PROGRAM MAIN

VAR CONSTANT
	cInitSourceFFT			: ST_MA_MultiArray_InitPars := ( eTypeCode := eMA_TypeCode_LREAL, nDims := 1, aDimSizes := [cFFTLength]);	
	cInitSourceSDFT			: ST_MA_MultiArray_InitPars := ( eTypeCode := eMA_TypeCode_LREAL, nDims := 1, aDimSizes := [cOversamples]);
	cInitParsSDFT			: ST_CM_SlidingDFT_InitPars := ( nWindowLength := cFFTLength, nBins := cBins, fDampingFactor := cDampingFactor);
END_VAR

VAR
	(* Input *)
	nInputSelection		: UDINT := 1;						// Switch between hardware and function generator	
	nSample				: UDINT;   
	aEl3632 AT %I*		: ARRAY[1..cOversamples] OF INT;	// Input from hardware e.g. EL3632
	
	(* Signal generation *)
	fbFunctionGenerator	: FB_FunctionGenerator;
	nSetFrequencyBin	: UDINT		:= 32;
	fSetFrequency		: LREAL 	:= nSetFrequencyBin * cResolution;	// Frequency of generated signal in Hz
	fSetAmplitude		: LREAL 	:= 5;								// peak amplitude OF SIN signal in Volts	
    fDC					: LREAL 	:= 1;       						// Amplitude of DC in Volts
	
	(* Source buffers *)	
	aBuffer				: ARRAY[1..cOversamples] OF LREAL;				// local varibale -> to source
	fbSourceFFT			: FB_CMA_Source :=(stInitPars := cInitSourceFFT, nOwnID := eID_SourceFFT, aDestIDs := [eID_FFT], nResultBuffers := 6);
	fbSourceSDFT		: FB_CMA_Source :=(stInitPars := cInitSourceSDFT, nOwnID := eID_SourceSDFT, aDestIDs := [eID_SDFT], nResultBuffers := 10);

	(* Sliding DFT *)
	bConfigured			: BOOL := FALSE;
	aConfParams			: ARRAY[1..cBins] OF UDINT;
	fbSlidingDFT		: FB_CMA_SlidingDFT := (stInitPars := cInitParsSDFT, nOwnID := eID_SDFT, aDestIDs := [eID_SinkSDFT]);
	
	(* Result buffers *)										
	aFFTResult			: ARRAY[1..cFFTResult] OF LCOMPLEX;				// local result variable <- from sink
	aSDFTResult			: ARRAY[1..cBins] OF LCOMPLEX;					// local result variable <- from sink
    
	(* Sinks *)
	fbSink_FFT			: FB_CMA_Sink := (nOwnID := eID_SinkFFT);		// Initialize sink buffers
	fbSink_SDFT			: FB_CMA_Sink := (nOwnID := eID_SinkSDFT);		// Initialize sink buffers
	
	(* post-processing of fft *)
	bCalculateFFT		: BOOL;											// true if fft calculation ready
	bCalculateSDFT		: BOOL;											// true if zoom fft calculation ready
	
	aSpectrumAbsFFT     : ARRAY[1..cFFTResult] OF LREAL; 				// magnitude spectrum
	aSpectrumFFTwin		: ARRAY[1..cFFTResult] OF LCOMPLEX;				// magnitude spectral bins
	aSpectrumAbsFFTwin	: ARRAY[1..cFFTResult] OF LREAL; 				// magnitude spectral bins
	
	aSpectrumAbsSDFT	: ARRAY[1..cBins] OF LREAL; 					// magnitude spectral bins
	aSpectrumSDFTwin	: ARRAY[1..cBins] OF LCOMPLEX;					// magnitude spectral bins
	aSpectrumAbsSDFTwin	: ARRAY[1..cBins] OF LREAL; 					// magnitude spectral bins
	
	(* error monitoring *)
	fbErrHist			: FB_HRErrHist;
END_VAR

(* Input *) 
CASE nInputSelection OF
	0:  (* input from EL3632 *)
		FOR nSample := 1 TO cOversamples DO
			aBuffer[nSample] := INT_TO_LREAL(aEl3632[nSample]);
		END_FOR
	1:  (* signal generator *)	
		fSetFrequency := nSetFrequencyBin * cResolution;
		fbFunctionGenerator(	fFrequency 	:= fSetFrequency,
								fAmplitude 	:= fSetAmplitude,
								eFunction 	:= E_FunctionType.Sine,
								aSignal		:= aBuffer );		
        // add DC to signal
		FOR nSample := 1 TO cOversamples DO
			aBuffer[nSample] := fDC + aBuffer[nSample];
		END_FOR								
END_CASE					

(* Call source to collect data *)
SourceBuffers();

(* Calculate Sliding DFT *)
CalculateSDFT();

(* Push results to sink *)
CollectFFT();

ACTION CalculateSDFT:
// Configure
IF NOT bConfigured THEN
	FOR nSample := 1 TO cBins DO
		aConfParams[nSample] := nSample - 1;
	END_FOR 
	fbSlidingDFT.Configure(pArg := ADR(aConfParams), nArgSize := SIZEOF(aConfParams));
	IF fbSlidingDFT.bError THEN
		fbErrHist.AddError(bErr:=TRUE, hrErrCode:=fbSlidingDFT.hrErrorCode, sErrSource:='MAIN.fbSlidingDFT.Configure'); // error monitoring
		// ToDo: if error
	ELSE
		bConfigured := TRUE;
	END_IF
END_IF

// Call SDFT 
fbSlidingDFT.Call();
IF fbSlidingDFT.bError THEN
	fbErrHist.AddError(bErr:=TRUE, hrErrCode:=fbSlidingDFT.hrErrorCode, sErrSource:='MAIN.fbSlidingDFT'); // error monitoring
	// ToDo: if error
END_IF

// Get SDFT
fbSink_SDFT.Output1DStd(pDataOut 		:= ADR(aSDFTResult), 
						nDataOutSize 	:= SIZEOF(aSDFTResult), 
						eElementType 	:= eMA_TypeCode_LCOMPLEX, 
						nOptionPars		:= 0,
						bNewResult		=> bCalculateSDFT);
IF fbSink_SDFT.bError THEN
	fbErrHist.AddError(bErr:=TRUE, hrErrCode:=fbSink_SDFT.hrErrorCode, sErrSource:='MAIN.fbSink_SDFT'); // error monitoring
	// ToDo: if error
END_IF

(* post-process fft result *)
IF bCalculateSDFT THEN
	// Calculate absolute value as aZoomFFTResult is of complex type
	FOR nSample := 1 TO cBins DO			   	   
	   	aSpectrumAbsSDFT[nSample] := SQRT(aSDFTResult[nSample].re * aSDFTResult[nSample].re + aSDFTResult[nSample].im * aSDFTResult[nSample].im);       
	   	// scale spectrum
		IF nSample = 1 THEN
			aSpectrumAbsSDFT[nSample] := (1.0 / cDampingFactor) * aSpectrumAbsSDFT[nSample] / cFFTLength ;   // scale DC value
		ELSE
			aSpectrumAbsSDFT[nSample] := (2.0 / cDampingFactor) * aSpectrumAbsSDFT[nSample] / cFFTLength; 	// scale frequencies not equal to 0
		END_IF
		
	END_FOR;
	
	// Apply Hanning window in frequency domain, i.e. X(k) = 0.5 * (-X(k-1) + 2 * X(k) - X(k+1)) 
	
	// DC
	aSpectrumSDFTwin[1].re := -aSDFTResult[cBins].re + 2 * aSDFTResult[1].re - aSDFTResult[2].re;
	aSpectrumSDFTwin[1].im := -aSDFTResult[cBins].im + 2 * aSDFTResult[1].re - aSDFTResult[2].im;
	aSpectrumAbsSDFTwin[1] := 0.5 * SQRT(aSpectrumSDFTwin[1].re * aSpectrumSDFTwin[1].re + aSpectrumSDFTwin[1].im * aSpectrumSDFTwin[1].im) / cFFTLength;
	FOR nSample := 2 TO cBins-1 DO	
		// Non-DC
		aSpectrumSDFTwin[nSample].re := -aSDFTResult[nSample - 1].re + 2 * aSDFTResult[nSample].re - aSDFTResult[nSample + 1].re;
		aSpectrumSDFTwin[nSample].im := -aSDFTResult[nSample - 1].im + 2 * aSDFTResult[nSample].im - aSDFTResult[nSample + 1].im;
		aSpectrumAbsSDFTwin[nSample] := SQRT(aSpectrumSDFTwin[nSample].re * aSpectrumSDFTwin[nSample].re + aSpectrumSDFTwin[nSample].im * aSpectrumSDFTwin[nSample].im) / cFFTLength;  
	END_FOR
END_IF
END_ACTION

ACTION CollectFFT:
// FFT
fbSink_FFT.Output1DStd(	pDataOut 		:= ADR(aFFTResult), 
						nDataOutSize 	:= SIZEOF(aFFTResult), 
						eElementType 	:= eMA_TypeCode_LCOMPLEX, 
						nOptionPars		:= 0,
						bNewResult		=> bCalculateFFT);
IF fbSink_FFT.bError THEN
	fbErrHist.AddError(bErr:=TRUE, hrErrCode:=fbSink_FFT.hrErrorCode, sErrSource:='MAIN.fbSink_FFT'); // error monitoring
	// ToDo: if error
END_IF

(* post-process fft result *)
IF bCalculateFFT THEN
	// Calculate absolute value as aFFTResult is of complex type
	FOR nSample := 1 TO cFFTResult DO			   	   
	   aSpectrumAbsFFT[nSample] := SQRT(aFFTResult[nSample].re * aFFTResult[nSample].re + aFFTResult[nSample].im * aFFTResult[nSample].im);       
	   // scale spectrum
	   IF nSample = 1 THEN
		   aSpectrumAbsFFT[nSample] := aSpectrumAbsFFT[nSample] / cFFTLength;   	// scale DC value
	   ELSE
		   aSpectrumAbsFFT[nSample] := 2 * aSpectrumAbsFFT[nSample] / cFFTLength; 	// scale frequencies not equal to 0
	   END_IF
	END_FOR;
	
	// Apply Hanning window in frequency domain, i.e. X(k) = 0.5 * (-X(k-1) + 2 * X(k) - X(k+1))
	
	// DC
	aSpectrumFFTwin[1].re := -aFFTResult[cBins].re + 2 * aFFTResult[1].re - aFFTResult[2].re;
	aSpectrumFFTwin[1].im := -aFFTResult[cBins].im + 2 * aFFTResult[1].re - aFFTResult[2].im;
	aSpectrumAbsFFTwin[1] := 0.5 * SQRT(aSpectrumFFTwin[1].re * aSpectrumFFTwin[1].re + aSpectrumFFTwin[1].im * aSpectrumFFTwin[1].im) / cFFTLength;
	FOR nSample := 2 TO cFFTResult-1 DO	
		// Non-DC
		aSpectrumFFTwin[nSample].re := -aFFTResult[nSample - 1].re + 2 * aFFTResult[nSample].re - aFFTResult[nSample + 1].re;
		aSpectrumFFTwin[nSample].im := -aFFTResult[nSample - 1].im + 2 * aFFTResult[nSample].im - aFFTResult[nSample + 1].im;
		aSpectrumAbsFFTwin[nSample] := SQRT(aSpectrumFFTwin[nSample].re * aSpectrumFFTwin[nSample].re + aSpectrumFFTwin[nSample].im * aSpectrumFFTwin[nSample].im) / cFFTLength;  
	END_FOR
END_IF
END_ACTION

ACTION SourceBuffers:
// FFT
fbSourceFFT.Input1DStd( pDataIn 		:= ADR(aBuffer),
						nDataInSize 	:= SIZEOF(aBuffer), 
						eElementType 	:= eMA_TypeCode_LREAL,
						nOptionPars		:= cCMA_Option_MarkInterruption );
IF fbSourceFFT.bError THEN
	fbErrHist.AddError(bErr:=TRUE, hrErrCode:=fbSourceFFT.hrErrorCode, sErrSource:='MAIN.fbSourceFFT'); // error monitoring
	// ToDo: if error
END_IF
 
// SDFT
fbSourceSDFT.Input1DStd( pDataIn 		:= ADR(aBuffer),
						nDataInSize 	:= SIZEOF(aBuffer), 
						eElementType 	:= eMA_TypeCode_LREAL,
						nOptionPars		:= cCMA_Option_MarkInterruption ); 
IF fbSourceSDFT.bError THEN
	fbErrHist.AddError(bErr:=TRUE, hrErrCode:=fbSourceSDFT.hrErrorCode, sErrSource:='MAIN.fbSourceSDFT'); // error monitoring
	// ToDo: if error
END_IF
END_ACTION

END_PROGRAM
